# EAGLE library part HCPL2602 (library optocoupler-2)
HEWLETT PACKARD OPTO COUPLER
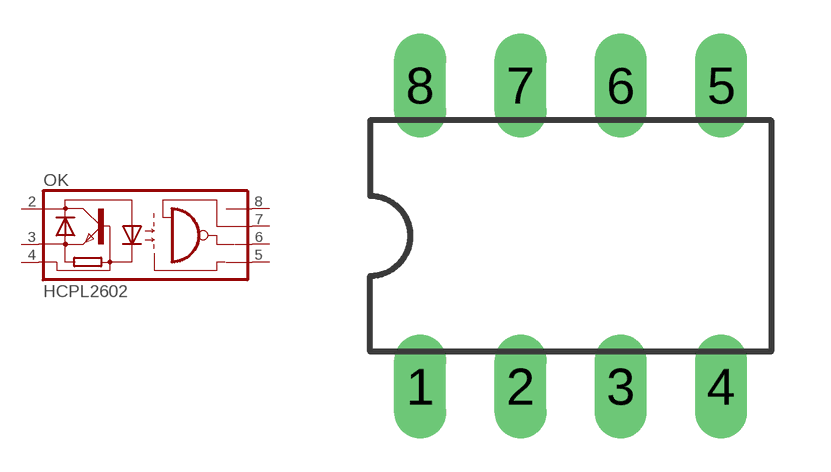
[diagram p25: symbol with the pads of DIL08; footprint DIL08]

Designator prefix OK

## HCPL2602  [DIL08]
2  +  pas
3  -  pas
4  B  pas
5  GND  pas
6  OUT  pas
7  EN  pas
8  VCC  pas

## Footprint DIL08 (pad centres in mm)
Dual In Line Package
drill 0.813 long: 1 -3.81,-3.81; 2 -1.27,-3.81; 3 1.27,-3.81; 4 3.81,-3.81; 5 3.81,3.81; 6 1.27,3.81; 7 -1.27,3.81; 8 -3.81,3.81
